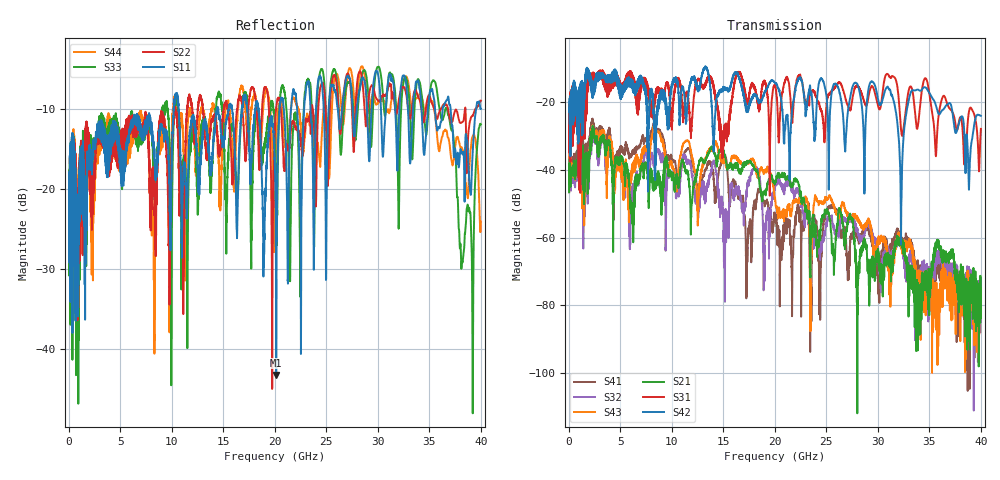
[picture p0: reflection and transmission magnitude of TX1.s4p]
!Agilent Technologies,N5245A,MY49151084,A.09.00.04
!Agilent N5245A: A.09.00.04
!Date: Thursday, January 20, 2011 08:53:15
!Correction: S11(Full 4 Port(1,2,3,4))
!S12(Full 4 Port(1,2,3,4))
!S13(Full 4 Port(1,2,3,4))
!S14(Full 4 Port(1,2,3,4))
!S21(Full 4 Port(1,2,3,4))
!S22(Full 4 Port(1,2,3,4))
!S23(Full 4 Port(1,2,3,4))
!S24(Full 4 Port(1,2,3,4))
!S31(Full 4 Port(1,2,3,4))
!S32(Full 4 Port(1,2,3,4))
!S33(Full 4 Port(1,2,3,4))
!S34(Full 4 Port(1,2,3,4))
!S41(Full 4 Port(1,2,3,4))
!S42(Full 4 Port(1,2,3,4))
!S43(Full 4 Port(1,2,3,4))
!S44(Full 4 Port(1,2,3,4))
!S4P File: Measurements: <S11,S12,S13,S14>,
!<S21,S22,S23,S24>,
!<S31,S32,S33,S34>,
!<S41,S42,S43,S44>:
# Hz S  dB  R 50
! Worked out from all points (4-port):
!   3996 points, 50 MHz to 40 GHz, reference 50 ohm
!   strongest paths, dB at 50 MHz, 10.04 GHz, 20.03 GHz, 30.02 GHz, 40 GHz:
!     S42: -22.8, -14.8, -14.3, -19.1, -24.1
!     S31: -22.8, -25.8, -15.3, -21.0, -27.9
!     S21: -46.6, -41.4, -43.6, -66.3, -76.5
!     S43: -46.5, -39.3, -48.1, -61.2, -82.9
!     S32: -46.7, -41.4, -44.5, -62.7, -82.0
!     S41: -45.3, -37.4, -55.1, -75.2, -71.9
!   lowest |S11| = -43.2 dB at 20.14 GHz (marker M1), VSWR 1.01, Z = 50.5 + j0.475 ohm
!   |S11| at or under -10 dB: start of sweep to 10.19 GHz; 10.67 GHz to 14.4 GHz (3.723 GHz wide, 29.7 % of centre); 37.07 GHz to 39.53 GHz (2.463 GHz wide, 6.43 % of centre)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
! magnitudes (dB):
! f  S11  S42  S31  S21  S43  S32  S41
! 50 MHz  -19.5  -22.8  -22.8  -46.6  -46.5  -46.7  -45.3
! 8.3 GHz  -15.9  -25.3  -20.8  -43.8  -27.6  -38.5  -27.1
! 20.14 GHz  -43.2  -14.5  -16.7  -42.4  -50.8  -43.9  -54.4
! 31.02 GHz  -6.4  -15.9  -11.9  -67.1  -69.8  -65.1  -66.1
! 32.26 GHz  -6.9  -56.0  -28.4  -61.0  -61.7  -60.2  -61.8
! 33.36 GHz  -11.5  -16.5  -16.6  -70.4  -62.9  -67.1  -64.0
! 40 GHz  -9.9  -24.1  -27.9  -76.5  -82.9  -82.0  -71.9
